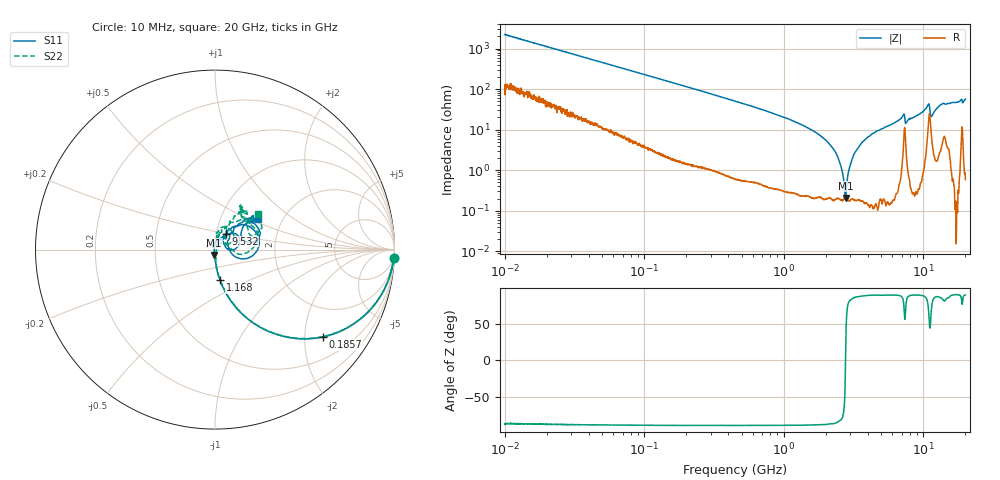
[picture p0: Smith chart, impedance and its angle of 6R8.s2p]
!Keysight Technologies,P5008B,MY61100088,A.16.20.02
!Date: Friday, August 30, 2024 13:15:21
!Correction: S11(C  2-Port  )
!S21(C  2-Port  )
!S12(C  2-Port  )
!S22(C  2-Port  )
!S2P File: Measurements: S11, S21, S12, S22:Log Frequency Sweep
# Hz S  dB  R 50
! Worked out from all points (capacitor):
!   1601 points, 10 MHz to 20 GHz, reference 50 ohm
!   read as one part in series: C = 7.15 pF near 10.39 MHz
!   lowest |Z| = 206 mohm at 2.772 GHz (marker M1)
!   series resonance near 2.767 GHz, so ESL is about 460 pH
!   S11 on the Smith chart (normalised r, x): 10 MHz: 3, -44; 185.7 MHz: 1.02, -2.47; 1.168 GHz: 1.00, -0.35; 9.532 GHz: 1.11, +0.20; 20 GHz: 1.51, +0.57
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1e7  -0.02 -2.6  -26.99 84.7  -26.99 84.8  -0.03 -2.6
3.555162e7  -0.14 -8.9  -16.23 79.4  -16.23 79.4  -0.15 -8.9
1.263918e8  -1.20 -28.8  -6.41 60.5  -6.42 60.5  -1.19 -28.7
1.857092e8  -2.22 -38.8  -4.12 50.6  -4.12 50.6  -2.22 -38.7
4.472136e8  -6.87 -63.0  -1.05 26.4  -1.06 26.4  -6.87 -62.8
1.167535e9  -15.25 -80.3  -0.16 8.6  -0.16 8.6  -15.25 -80.7
1.589917e9  -18.98 -84.8  -0.07 4.6  -0.08 4.6  -18.96 -84.0
2.30303e9  -25.16 -89.6  -0.03 0.3  -0.03 0.3  -24.99 -86.1
2.771802e9  -30.41 -97.8  -0.02 -1.8  -0.02 -1.8  -29.88 -78.0
3.048071e9  -34.81 -104.0  -0.02 -2.9  -0.02 -3.0  -33.61 -71.4
3.465213e9  -45.83 -173.0  -0.01 -4.5  -0.01 -4.5  -40.56 -19.5
3.616581e9  -42.13 102.9  -0.01 -5.0  -0.01 -5.1  -41.37 37.4
3.846973e9  -35.65 114.9  -0.01 -5.8  -0.01 -5.9  -34.99 42.6
4.270791e9  -30.64 93.0  -0.01 -7.2  -0.01 -7.3  -30.40 66.0
5.652411e9  -26.20 78.1  -0.01 -11.6  -0.01 -11.7  -25.61 73.3
7.100103e9  -18.40 47.5  -0.19 -17.6  -0.20 -17.7  -18.57 76.9
7.733948e9  -23.52 52.7  -0.08 -15.8  -0.08 -15.9  -23.68 74.8
9.531902e9  -19.37 56.2  -0.06 -23.1  -0.06 -23.2  -19.48 69.6
1.073392e10  -12.84 35.1  -0.82 -30.7  -0.82 -30.9  -12.86 46.3
1.169216e10  -21.36 34.2  -0.28 -23.5  -0.28 -23.7  -21.33 46.6
1.361179e10  -11.42 40.7  -0.60 -32.9  -0.60 -33.1  -11.38 54.6
2e10  -10.53 35.5  -0.45 -51.4  -0.45 -51.6  -10.21 39.4
